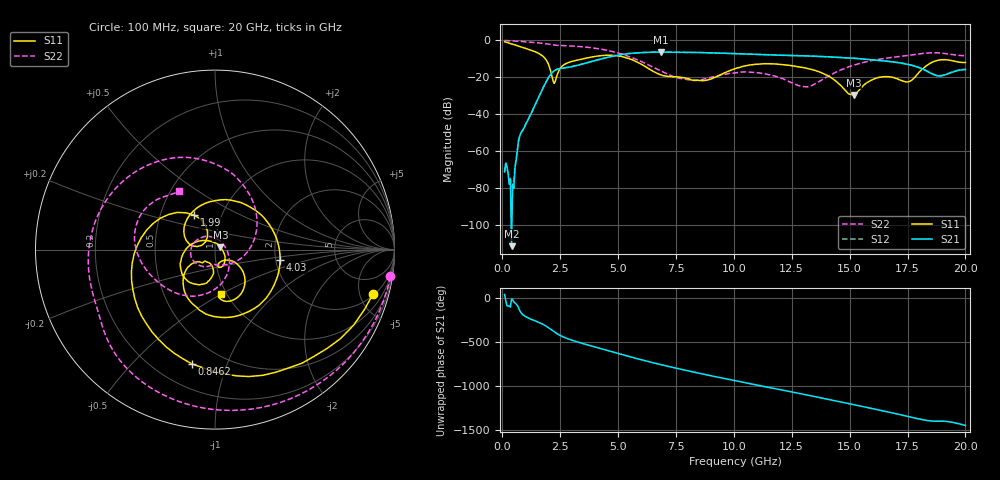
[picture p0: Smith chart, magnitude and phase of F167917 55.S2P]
!  2-Port S-parameters saved by WinCal
! VAR MeasName=S-Parameters (CALIBRATED_DATA) read from VNA (N5242A)
! VAR MeasDate=2016-11-22 9:02:39
! VAR NAME=F167917 55
! VAR FILENAME=F167917 55.S2P
! VAR DATE=2016-11-22 9:02:39
! VAR PHYS_PORTS=1,2
# Hz S DB R 50
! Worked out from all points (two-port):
!   401 points, 100 MHz to 20 GHz, reference 50 ohm
!   highest |S21| = -6.39 dB at 6.866 GHz (marker M1); lowest = -111.5 dB at 398.5 MHz (marker M2)
!   |S21| within 3 dB of the highest: 4.496 GHz to 14.73 GHz (10.24 GHz wide, 106 % of centre)
!   lowest |S11| = -29.6 dB at 15.17 GHz (marker M3), VSWR 1.07, Z = 53.1 + j1.47 ohm
!   |S11| at or under -10 dB: 1.855 GHz to 3.511 GHz (1.655 GHz wide, 61.7 % of centre); 5.493 GHz to end of sweep
!   |S22| runs from -25.2 to -0.1 dB; largest |S21 - S12| = 0.0039
!   S11 on the Smith chart (normalised r, x): 100 MHz: 2.17, -6.62; 846.2 MHz: 0.34, -0.76; 1.99 GHz: 0.74, +0.30; 4.03 GHz: 2.11, -0.28; 20 GHz: 0.94, -0.50
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1e8  -0.76 -15.6  -70.95 43.9  -71.80 45.3  -0.10 -8.7
3.985e8  -1.97 -52.5  -111.51 -12.5  -79.30 -50.1  -0.29 -32.9
8.4625e8  -3.74 -101.3  -49.39 -174.1  -49.48 -174.2  -0.67 -66.8
1.44325e9  -6.34 -165.1  -34.33 101.8  -34.30 101.8  -1.27 -106.7
1.9905e9  -12.93 121.3  -20.28 26.9  -20.25 27.0  -2.08 -138.6
2.23925e9  -23.35 142.6  -16.57 -20.3  -16.54 -20.1  -2.58 -150.1
2.63725e9  -13.47 144.4  -15.02 -80.1  -15.00 -80.1  -2.89 -166.7
3.43325e9  -10.24 50.1  -12.94 -151.6  -12.93 -151.6  -3.49 157.7
4.03025e9  -8.69 -9.1  -10.87 163.5  -10.86 163.7  -4.35 130.2
5.32375e9  -9.44 -107.4  -7.41 68.4  -7.37 68.3  -8.18 65.9
6.7665e9  -18.34 -145.9  -6.39 -30.4  -6.39 -30.5  -16.13 -16.8
6.866e9  -18.80 -143.8  -6.39 -36.7  -6.39 -36.8  -16.76 -22.8
8.10975e9  -21.13 -132.1  -6.59 -110.8  -6.58 -110.8  -21.42 -87.5
9.055e9  -20.71 -100.2  -6.85 -164.5  -6.84 -164.6  -19.96 -112.2
1.005e10  -15.44 -99.6  -7.21 141.6  -7.20 141.7  -17.65 -145.5
1.139325e10  -12.70 -132.3  -7.88 70.7  -7.82 70.7  -18.26 160.7
1.338325e10  -15.89 178.6  -8.58 -33.9  -8.57 -34.1  -24.41 9.0
1.517425e10  -29.58 24.6  -9.68 -131.5  -9.73 -131.5  -13.49 -86.9
1.67165e10  -19.80 -76.5  -11.47 141.6  -11.52 142.0  -9.46 -137.3
1.756225e10  -22.39 -55.0  -13.19 91.1  -13.12 91.5  -8.13 -161.0
1.885575e10  -10.72 -62.7  -19.30 39.6  -19.16 40.3  -6.83 153.3
2e10  -11.99 -82.5  -15.81 -9.0  -15.68 -9.0  -8.37 121.7
